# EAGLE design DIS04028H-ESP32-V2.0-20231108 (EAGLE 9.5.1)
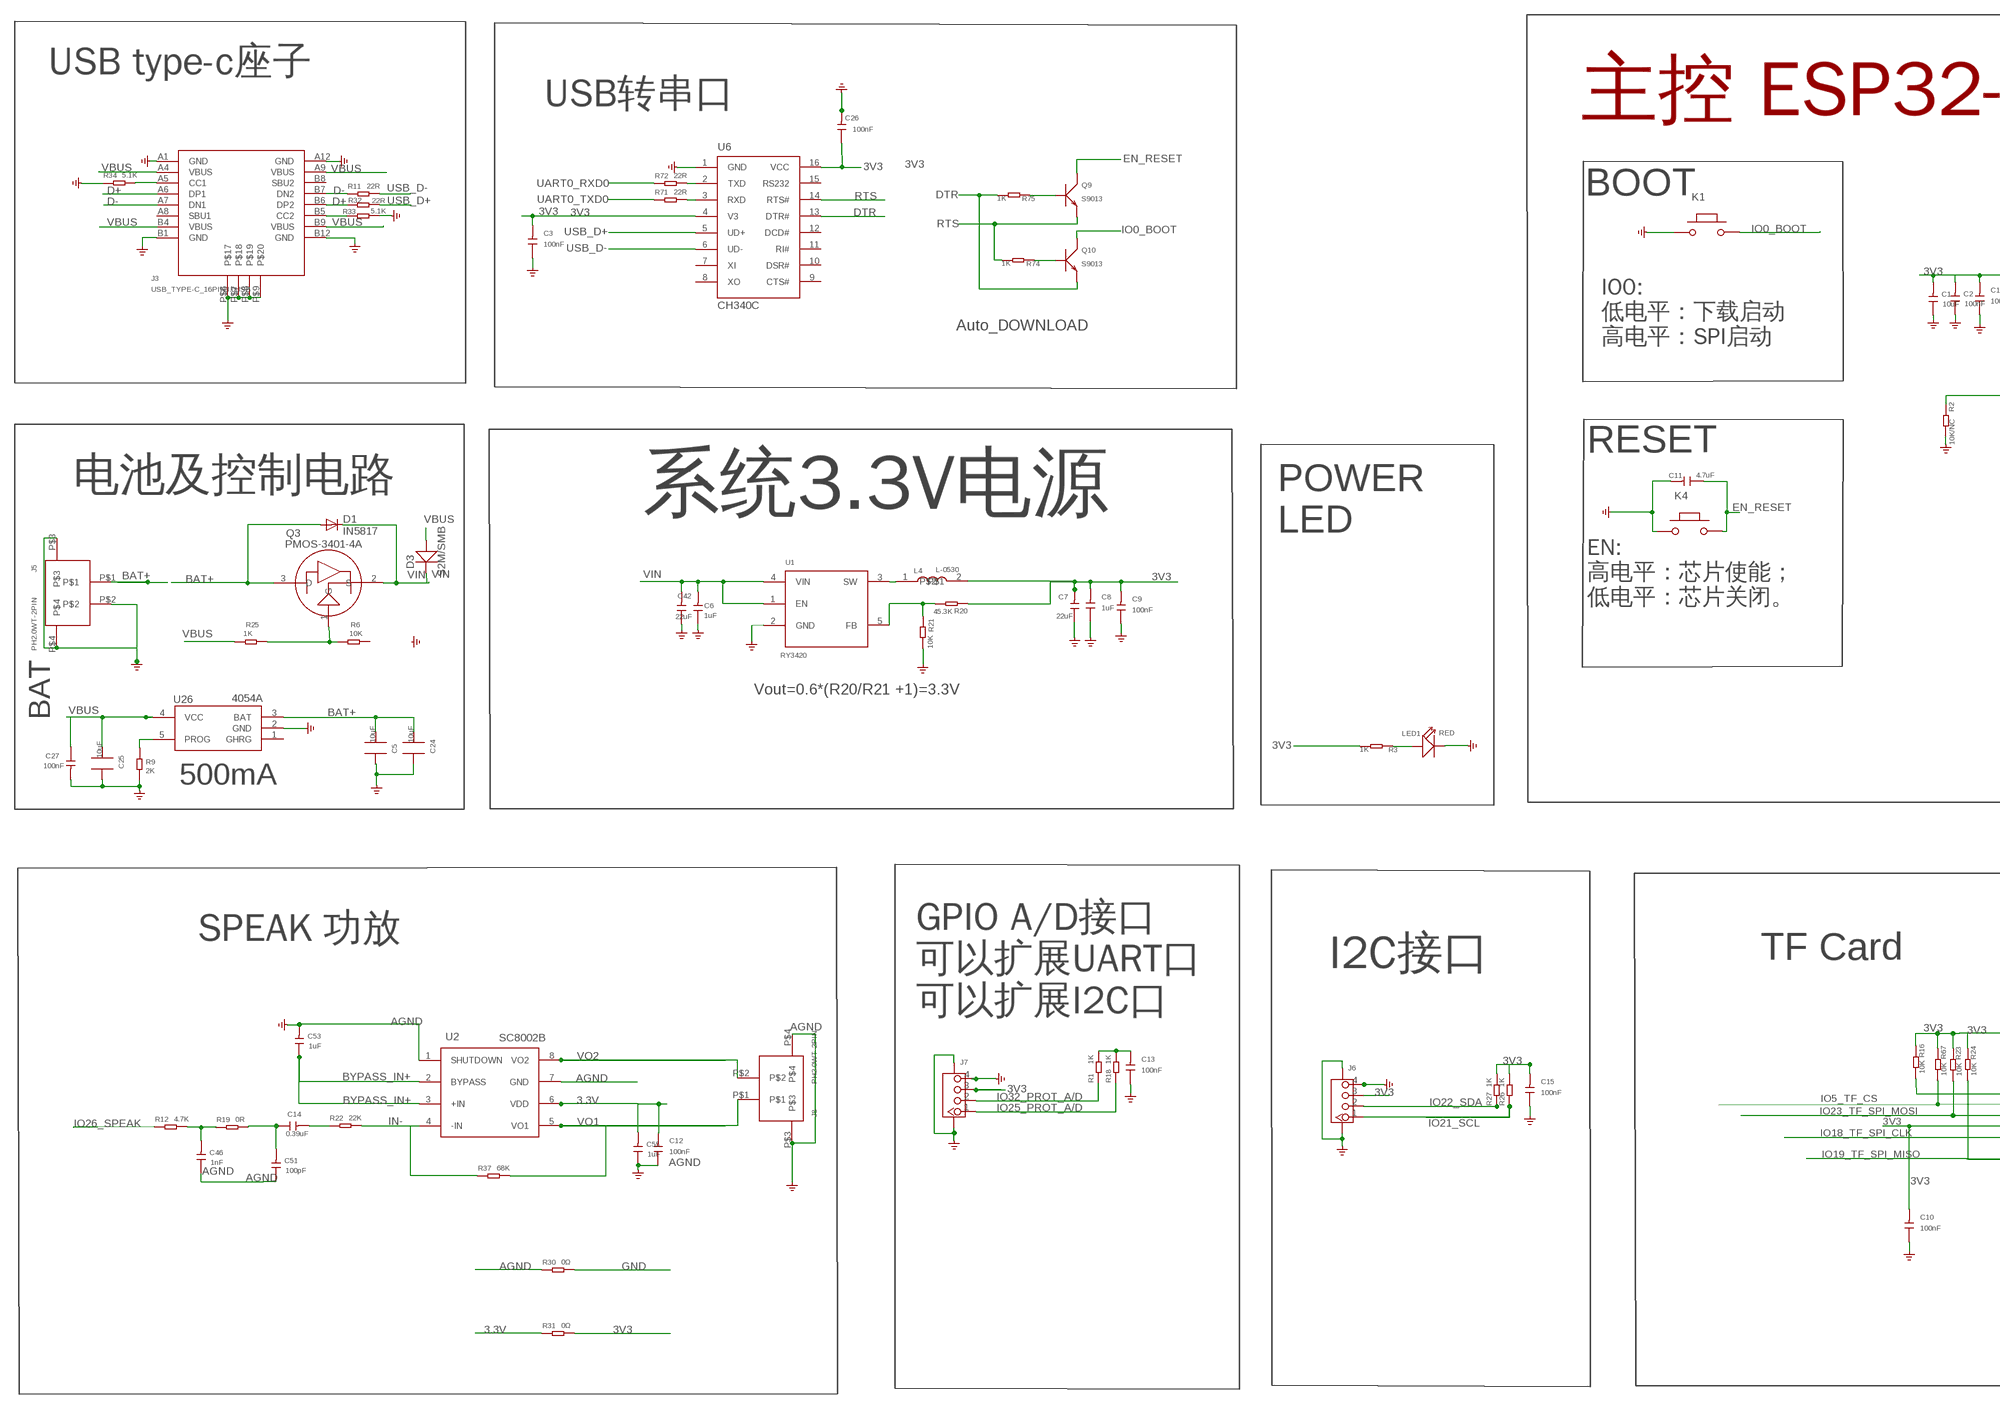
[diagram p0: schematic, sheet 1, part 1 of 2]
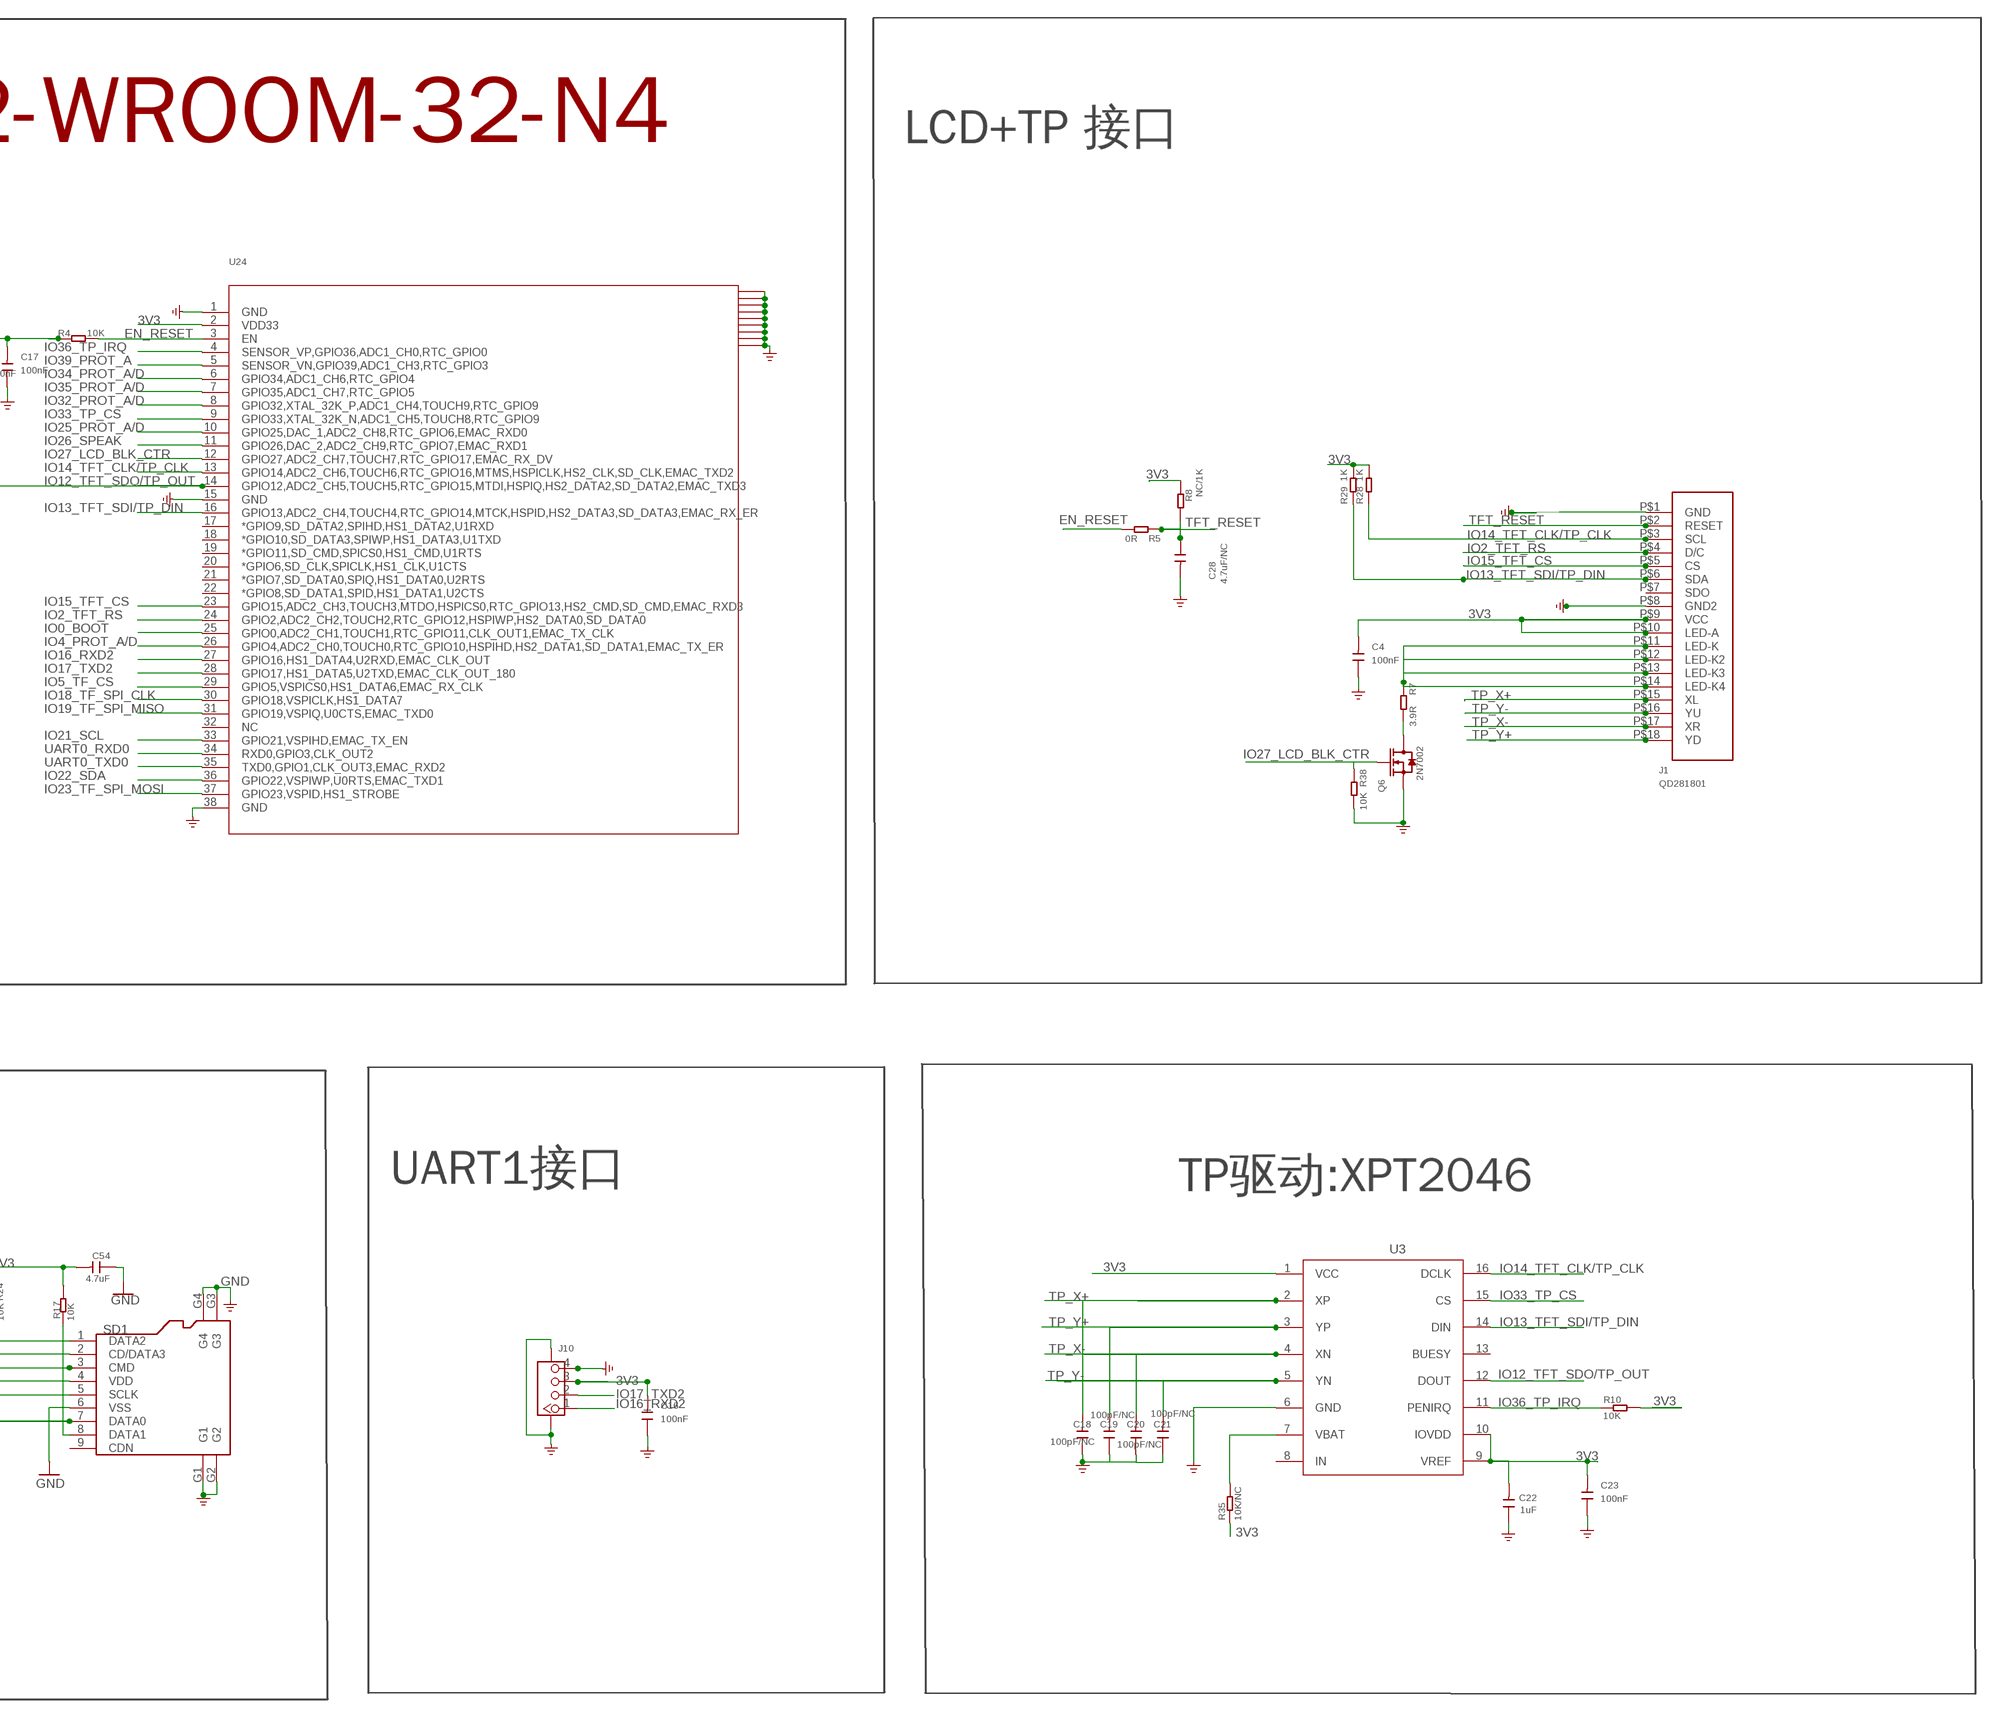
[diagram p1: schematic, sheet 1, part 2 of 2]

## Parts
C1  10uF  DISCRETE_C-0603  [DISCRETE_C0603]
C2  100nF  DISCRETE_C-0603  [DISCRETE_C0603]
C3  100nF  C0603  [0603]
C4  100nF  C0603  [0603]
C5  10uF  C0805_S  [0805_S]
C6  1uF  C0603  [0603]
C7  22uF  C0805  [0805]
C8  1uF  C0603  [0603]
C9  100nF  C0603  [0603]
C10  100nF  C0603  [0603]
C11  4.7uF  C0603  [0603]
C12  100nF  C0603  [0603]
C13  100nF  C0603  [0603]
C14  0.39uF  DISCRETE_C-0603  [DISCRETE_C0603]
C15  100nF  C0603  [0603]
C16  100nF  C0603  [0603]
C17  100nF  C0603  [0603]
C18  100pF/NC  C0603  [0603]
C19  100pF/NC  C0603  [0603]
C20  100pF/NC  C0603  [0603]
C21  100pF/NC  C0603  [0603]
C22  1uF  DISCRETE_C-0603  [DISCRETE_C0603]
C23  100nF  C0603  [0603]
C24  10uF  C0805_S  [0805_S]
C25  10uF  C0805_S  [0805_S]
C26  100nF  C0603  [0603]
C27  100nF  C-0603  [C0603]
C28  4.7uF/NC  C0603  [0603]
C42  22uF  C0805  [0805]
C46  1nF  DISCRETE_C-0603  [DISCRETE_C0603]
C51  100pF  DISCRETE_C-0603  [DISCRETE_C0603]
C53  1uF  DISCRETE_C-0603  [DISCRETE_C0603]
C54  4.7uF  DISCRETE_C-0603  [DISCRETE_C0603]
C55  1uF  DISCRETE_C-0603  [DISCRETE_C0603]
D1  IN5817  DIODE-DO-214AC  [DO-214AC]
D3  S2M/SMB  214ABDO-214AB  [214AB]
J1  QD281801  [QD241801-18PIN*0.8]
J3  USB_TYPE-C_16PIN3.0USB  [KEVIN_3.0TYPEC-SMD]
J5  PH2.0WT-2PIN  [PH2.0WT-2PIN]
J6  CONNECTOR_TWIG-4P-2.0-SMD-FEMALE-REINFORCE90D  [CONNECTOR_4P-SMD-2.0-90D]
J7  CONNECTOR_TWIG-4P-2.0-SMD-FEMALE-REINFORCE90D  [CONNECTOR_4P-SMD-2.0-90D]
J8  PH2.0WT-2PIN  [PH2.0WT-2PIN]
J10  CONNECTOR_TWIG-4P-2.0-SMD-FEMALE-REINFORCE90D  [CONNECTOR_4P-SMD-2.0-90D]
K1  BUTTON  PB157  [157SW]
K4  BUTTON  PB157  [157SW]
L4  L-0530  [CD54_CD54]
LED1  RED  DISCRETE_LED0603  [DISCRETE_LED-0603]
Q3  PMOS-3401-4A  P-MOS-SOT23  [SOT-23]
Q6  2N7002  MOSFET-N'SOT23'  [SOT23]
Q9  S9013  TRANSISTOR-NPN-SOT23  [SOT23@1]
Q10  S9013  TRANSISTOR-NPN-SOT23  [SOT23@1]
R1  1K  DISCRETE_R-0603  [DISCRETE_R0603]
R2  10K/NC  DISCRETE_R-0603  [DISCRETE_R0603]
R3  1K  DISCRETE_R-0603  [DISCRETE_R0603]
R4  10K  R0603  [R0603]
R5  0R  DISCRETE_R-0603  [DISCRETE_R0603]
R6  10K  DISCRETE_R-0603  [DISCRETE_R0603]
R7  3.9R  DISCRETE_R-0603  [DISCRETE_R0603]
R8  NC/1K  DISCRETE_R-0603  [DISCRETE_R0603]
R9  2K  DISCRETE_R-0603  [DISCRETE_R0603]
R10  10K  DISCRETE_R-0603  [DISCRETE_R0603]
R11  22R  DISCRETE_R-0603  [DISCRETE_R0603]
R12  4.7K  DISCRETE_R-0603  [DISCRETE_R0603]
R16  10K  DISCRETE_R-0603  [DISCRETE_R0603]
R17  10K  DISCRETE_R-0603  [DISCRETE_R0603]
R18  1K  DISCRETE_R-0603  [DISCRETE_R0603]
R19  0R  DISCRETE_R-0603  [DISCRETE_R0603]
R20  45.3K  DISCRETE_R-0603  [DISCRETE_R0603]
R21  10K  DISCRETE_R-0603  [DISCRETE_R0603]
R22  22K  DISCRETE_R-0603  [DISCRETE_R0603]
R23  10K  DISCRETE_R-0603  [DISCRETE_R0603]
R24  10K  DISCRETE_R-0603  [DISCRETE_R0603]
R25  1K  DISCRETE_R-0603  [DISCRETE_R0603]
R26  1K  DISCRETE_R-0603  [DISCRETE_R0603]
R27  1K  DISCRETE_R-0603  [DISCRETE_R0603]
R28  1K  DISCRETE_R-0603  [DISCRETE_R0603]
R29  1K  DISCRETE_R-0603  [DISCRETE_R0603]
R30  0Ω  DISCRETE_R-0603  [DISCRETE_R0603]
R31  0Ω  DISCRETE_R-0603  [DISCRETE_R0603]
R32  22R  DISCRETE_R-0603  [DISCRETE_R0603]
R33  5.1K  DISCRETE_R-0603  [DISCRETE_R0603]
R34  5.1K  DISCRETE_R-0603  [DISCRETE_R0603]
R35  10K/NC  DISCRETE_R-0603  [DISCRETE_R0603]
R37  68K  DISCRETE_R-0603  [DISCRETE_R0603]
R38  10K  DISCRETE_R-0603  [DISCRETE_R0603]
R67  10K  DISCRETE_R-0603  [DISCRETE_R0603]
R71  22R  DISCRETE_R-0603  [DISCRETE_R0603]
R72  22R  DISCRETE_R-0603  [DISCRETE_R0603]
R74  1K  DISCRETE_R-0603  [DISCRETE_R0603]
R75  1K  DISCRETE_R-0603  [DISCRETE_R0603]
SD1  HOLDER-MICROSD-9P  [9P-SMD-W/-RING]
U1  RY3420  A_XBJ_HM3420B  [A_XBJ_SOT23-5]
U2  SC8002B  SC8002BSC8002B-SOP8  [AT24C02_SOP8]
U3  XP2046  [XP2046-SSOP16]
U6  CH340C  CH340G  [SOP-16]
U24  ESP32-WROOM-32-N4  [ESP32-WROOM-32-N4]
U26  4054A  [SOP23-5]

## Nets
3.3V: C12.2 C55.2 R31.1 U2.6(VDD)
3V3: C1.2 C2.2 C3.2 C4.2 C7.2 C8.2 C9.2 C10.2 C13.2 C15.2 C16.2 C17.2 C22.2 C23.2 C26.1 C54.2 J1.P$9(VCC) J1.P$10(LED-A) J6.3 J7.3 J10.3 L4.2 R1.2 R3.2 R4.1 R8.2 R10.2 R16.1 R17.1 R18.2 R20.1 R23.1 R24.1 R26.2 R27.2 R28.2 R29.2 R31.2 R35.1 R67.1 SD1.4(VDD) U3.1(VCC) U3.9(VREF) U3.10(IOVDD) U6.4(V3) U6.16(VCC) U24.2(VDD33)
AGND: C12.1 C46.1 C51.1 C53.2 C55.1 J8.P$3 J8.P$4 R30.1 U2.1(SHUTDOWN) U2.7(GND) ; supply symbol labelled GND
BAT+: C5.2 C24.2 D1.A J5.P$1 Q3.3(D) U26.3(BAT)
BYPASS_IN+: C53.1 U2.2(BYPASS) U2.3(+IN)
D+: J3.A6(DP1) J3.B6(DP2) R32.1
D-: J3.A7(DN1) J3.B7(DN2) R11.1
DTR: Q10.2(E) R75.2 U6.13(DTR#)
EN_RESET: C11.1 K4.2 Q9.3(C) R4.2 R5.2 U24.3(EN)
GND: C1.1 C2.1 C3.1 C4.1 C5.1 C6.1 C7.1 C8.1 C9.1 C10.1 C11.2 C13.1 C15.1 C16.1 C17.1 C18.1 C19.1 C20.1 C21.1 C22.1 C23.1 C24.1 C25.1 C26.2 C27.2 C28.2 C42.1 C54.1 J1.P$1(GND) J1.P$8(GND2) J3.A1(GND) J3.A12(GND) J3.B1(GND) J3.B12(GND) J3.P$6 J3.P$7 J3.P$8 J3.P$9 J5.P$2 J5.P$3 J5.P$4 J6.4 J6.SS1 J6.SS2 J7.4 J7.SS1 J7.SS2 J10.4 J10.SS1 J10.SS2 K1.1 K4.1 LED1.- Q6.2(S) R2.2 R9.2 R21.2 R30.2 R33.2 R34.1 R38.2 SD1.6(VSS) SD1.G1 SD1.G2 SD1.G3 SD1.G4 U1.2(GND) U3.6(GND) U6.1(GND) U24.1(GND) U24.15(GND) U24.38(GND) U24.41(GND) U24.42(GND) U24.43(GND) U24.44(GND) U24.45(GND) U24.46(GND) U24.47(GND) U24.48(GND) U24.49(GND) U26.2(GND)
IN-: R22.2 R37.1 U2.4(-IN)
IO0_BOOT: K1.2 Q10.3(C) U24.25(GPIO0,ADC2_CH1,TOUCH1,RTC_GPIO11,CLK_OUT1,EMAC_TX_CLK)
IO2_TFT_RS: J1.P$4(D/C) U24.24(GPIO2,ADC2_CH2,TOUCH2,RTC_GPIO12,HSPIWP,HS2_DATA0,SD_DATA0)
IO4_PROT_A/D: U24.26(GPIO4,ADC2_CH0,TOUCH0,RTC_GPIO10,HSPIHD,HS2_DATA1,SD_DATA1,EMAC_TX_ER)
IO5_TF_CS: R67.2 SD1.2(CD/DATA3) U24.29(GPIO5,VSPICS0,HS1_DATA6,EMAC_RX_CLK)
IO12_TFT_SDO/TP_OUT: R2.1 U3.12(DOUT) U24.14(GPIO12,ADC2_CH5,TOUCH5,RTC_GPIO15,MTDI,HSPIQ,HS2_DATA2,SD_DATA2,EMAC_TXD3)
IO13_TFT_SDI/TP_DIN: J1.P$6(SDA) R29.1 U3.14(DIN) U24.16(GPIO13,ADC2_CH4,TOUCH4,RTC_GPIO14,MTCK,HSPID,HS2_DATA3,SD_DATA3,EMAC_RX_ER)
IO14_TFT_CLK/TP_CLK: J1.P$3(SCL) R28.1 U3.16(DCLK) U24.13(GPIO14,ADC2_CH6,TOUCH6,RTC_GPIO16,MTMS,HSPICLK,HS2_CLK,SD_CLK,EMAC_TXD2)
IO15_TFT_CS: J1.P$5(CS) U24.23(GPIO15,ADC2_CH3,TOUCH3,MTDO,HSPICS0,RTC_GPIO13,HS2_CMD,SD_CMD,EMAC_RXD3)
IO16_RXD2: J10.1 U24.27(GPIO16,HS1_DATA4,U2RXD,EMAC_CLK_OUT)
IO17_TXD2: J10.2 U24.28(GPIO17,HS1_DATA5,U2TXD,EMAC_CLK_OUT_180)
IO18_TF_SPI_CLK: SD1.5(SCLK) U24.30(GPIO18,VSPICLK,HS1_DATA7)
IO19_TF_SPI_MISO: R24.2 SD1.7(DATA0) U24.31(GPIO19,VSPIQ,U0CTS,EMAC_TXD0)
IO21_SCL: J6.1 R26.1 U24.33(GPIO21,VSPIHD,EMAC_TX_EN)
IO22_SDA: J6.2 R27.1 U24.36(GPIO22,VSPIWP,U0RTS,EMAC_TXD1)
IO23_TF_SPI_MOSI: R23.2 SD1.3(CMD) U24.37(GPIO23,VSPID,HS1_STROBE)
IO25_PROT_A/D: J7.1 R18.1 U24.10(GPIO25,DAC_1,ADC2_CH8,RTC_GPIO6,EMAC_RXD0)
IO26_SPEAK: R12.1 U24.11(GPIO26,DAC_2,ADC2_CH9,RTC_GPIO7,EMAC_RXD1)
IO27_LCD_BLK_CTR: Q6.1(G) R38.1 U24.12(GPIO27,ADC2_CH7,TOUCH7,RTC_GPIO17,EMAC_RX_DV)
IO32_PROT_A/D: J7.2 R1.1 U24.8(GPIO32,XTAL_32K_P,ADC1_CH4,TOUCH9,RTC_GPIO9)
IO33_TP_CS: U3.15(CS) U24.9(GPIO33,XTAL_32K_N,ADC1_CH5,TOUCH8,RTC_GPIO9)
IO34_PROT_A/D: U24.6(GPIO34,ADC1_CH6,RTC_GPIO4)
IO35_PROT_A/D: U24.7(GPIO35,ADC1_CH7,RTC_GPIO5)
IO36_TP_IRQ: R10.1 U3.11(PENIRQ) U24.4(SENSOR_VP,GPIO36,ADC1_CH0,RTC_GPIO0)
IO39_PROT_A: U24.5(SENSOR_VN,GPIO39,ADC1_CH3,RTC_GPIO3)
N$1: LED1.+ R3.1
N$2: Q6.3(D) R7.2
N$3: C46.2 R12.2 R19.1
N$4: R35.2 U3.7(VBAT)
N$6: R9.1 U26.5(PROG)
N$8: L4.1 U1.3(SW)
N$12: J1.P$11(LED-K) J1.P$12(LED-K2) J1.P$13(LED-K3) J1.P$14(LED-K4) R7.1
N$14: J3.B5(CC2) R33.1
N$16: J3.A5(CC1) R34.2
N$17: Q3.1(G) R6.2 R25.1
N$20: R20.2 R21.1 U1.5(FB)
N$26: C14.1 C51.2 R19.2
N$29: C14.2 R22.1
N$32: Q9.1(B) R75.1
N$38: Q10.1(B) R74.1
N$40: R72.2 U6.2(TXD)
N$42: R71.2 U6.3(RXD)
N$47: R16.2 SD1.1(DATA2)
N$48: R17.2 SD1.8(DATA1)
RTS: Q9.2(E) R74.2 U6.14(RTS#)
TFT_RESET: C28.1 J1.P$2(RESET) R5.1 R8.1
TP_X+: C18.2 J1.P$15(XL) U3.2(XP)
TP_X-: C20.2 J1.P$17(XR) U3.4(XN)
TP_Y+: C19.2 J1.P$18(YD) U3.3(YP)
TP_Y-: C21.2 J1.P$16(YU) U3.5(YN)
UART0_RXD0: R72.1 U24.34(RXD0,GPIO3,CLK_OUT2)
UART0_TXD0: R71.1 U24.35(TXD0,GPIO1,CLK_OUT3,EMAC_RXD2)
USB_D+: R32.2 U6.5(UD+)
USB_D-: R11.2 U6.6(UD-)
VBUS: C25.2 C27.1 D3.1(+) J3.A4(VBUS) J3.A9(VBUS) J3.B4(VBUS) J3.B9(VBUS) R25.2 U26.4(VCC)
VIN: C6.2 C42.2 D1.C D3.2(-) Q3.2(S) U1.1(EN) U1.4(VIN)
VO1: J8.P$1 R37.2 U2.5(VO1)
VO2: J8.P$2 U2.8(VO2)
Unconnected: J1.P$7(SDO) J3.A8(SBU1) J3.B8(SBU2) R6.1 SD1.9(CDN) U3.8(IN) U3.13(BUESY) U6.7(XI) U6.8(XO) U6.9(CTS#) U6.10(DSR#) U6.11(RI#) U6.12(DCD#) U6.15(RS232) U24.17(*GPIO9,SD_DATA2,SPIHD,HS1_DATA2,U1RXD) U24.18(*GPIO10,SD_DATA3,SPIWP,HS1_DATA3,U1TXD) U24.19(*GPIO11,SD_CMD,SPICS0,HS1_CMD,U1RTS) U24.20(*GPIO6,SD_CLK,SPICLK,HS1_CLK,U1CTS) U24.21(*GPIO7,SD_DATA0,SPIQ,HS1_DATA0,U2RTS) U24.22(*GPIO8,SD_DATA1,SPID,HS1_DATA1,U2CTS) U24.32(NC) U26.1(GHRG)

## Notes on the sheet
- USB type-c座子
- USB转串口 | 主控 ESP32-WROOM-32-N4 | LCD+TP 接口
- BOOT
- Auto_DOWNLOAD
- IO0:
  低电平：下载启动
  高电平：SPI启动
- RESET
- 电池及控制电路
- 系统3.3V电源
- POWER
  LED
- EN:
  高电平：芯片使能；
  低电平：芯片关闭。
- Vout=0.6*(R20/R21 +1)=3.3V
- BAT
- 500mA
- SPEAK 功放
- I2C接口 | TF Card | UART1接口
- TP驱动:XPT2046
- GPIO A/D接口
  可以扩展UART口
  可以扩展I2C口

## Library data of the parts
C1 C2 C14 C22 C46 C51 C53 C55 = A_xbj:DISCRETE_C*: Ceramic Capacitors
C3 C4 C6 C8-C13 C15-C21 C23 C26 C28 = A_xbj:C0603
C5 C24 C25 = CPT_SMD:C0805
C7 C42 = A_xbj:C0805
C27 = discrete:C*: Ceramic Capacitors
C54 = A9G:DISCRETE_C*: Ceramic Capacitors
D1 = diode:DIODE-: DIODE
D3 = DO-214AB:214AB: 214AB
J1 = cooper:QD281801
J3 = WZ3532R024-ESP32-V0.1-20221226:USB_TYPE-C_16PIN
J5 J8 = cooper:PH2.0WT-2PIN
J6 J7 J10 = A_xbj:CONNECTOR_TWIG-4P-2.0-SMD-FEMALE-REINFORCE
K1 K4 = MySMD:PB157
L4 = WZ2432R028-ESP32-V1.2-20231108:L-0530
LED1 = A_xbj:DISCRETE_LED*
Q3 = DFN8:P-MOS-SOT23
Q6 = discrete:MOSFET-N: IRLL014: http://www.vishay.com/docs/91319/sihll014.pdf
Q9 Q10 = discrete:TRANSISTOR-NPN*: NPN audion
R1-R3 R5 R7 R8 R11 R12 R16-R24 R26-R34 R37 R38 R67 R71 R72 R74 R75 = Crowtail-_LED-V2.0-20190615-01:DISCRETE_R*
R4 = A_xbj:R0603
R6 R9 R10 R25 R35 = A9G:DISCRETE_R*
SD1 = Connector:HOLDER-MICROSD-9P
U1 = CrowBot_-V1.0-20220525:A_XBJ_HM3420B
U2 = cooper:SC8002B
U3 = cooper:XP2046
U6 = A_xbj:CH340G
U24 = cooper:ESP32-WROOM-32-N4
U26 = DFN8:4054A

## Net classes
0 default: width 0.152 mm, drill 0.305 mm, clearance 0.203 mm

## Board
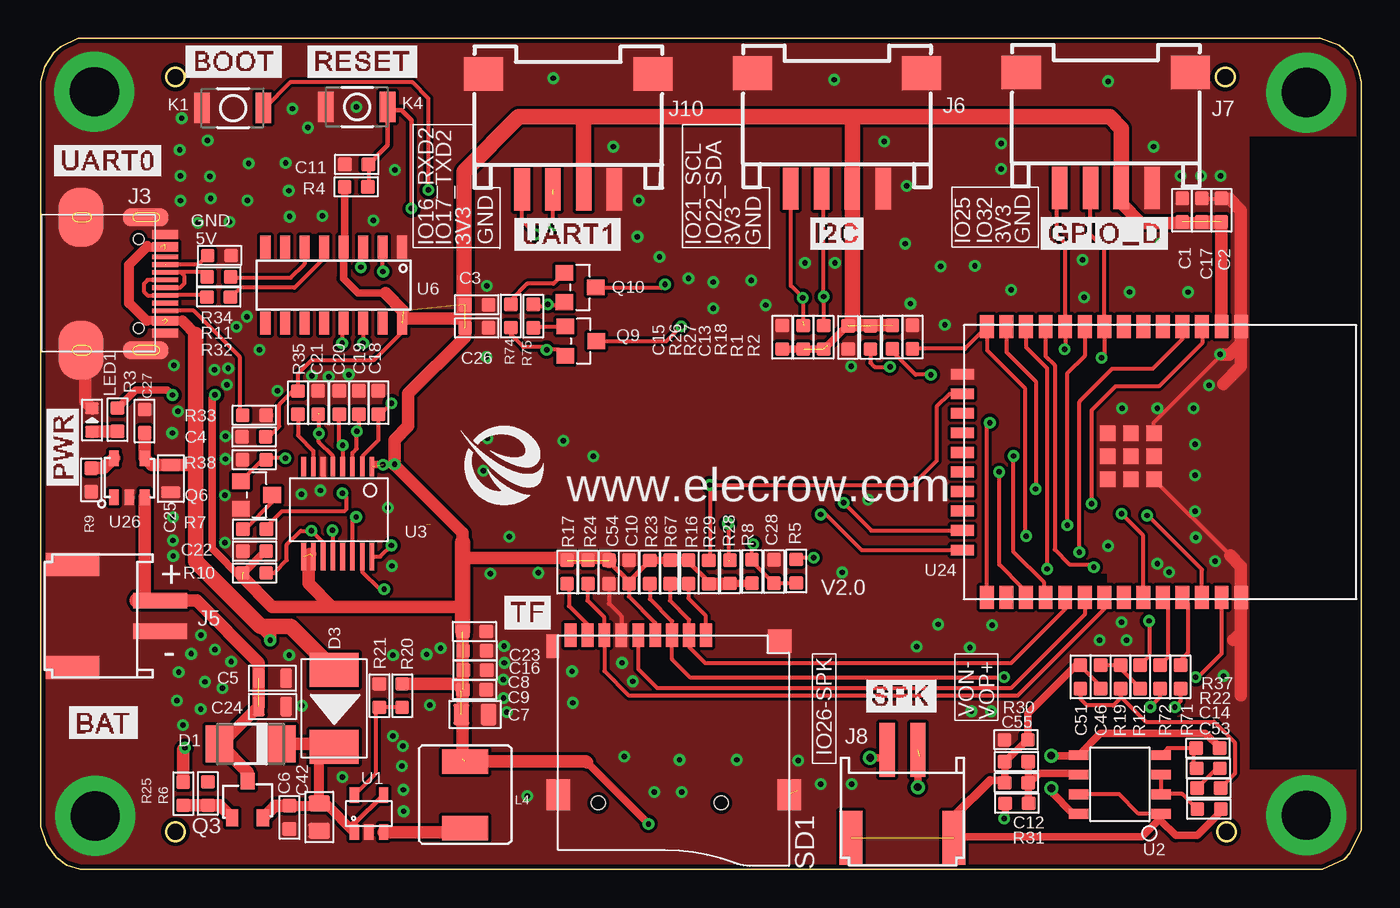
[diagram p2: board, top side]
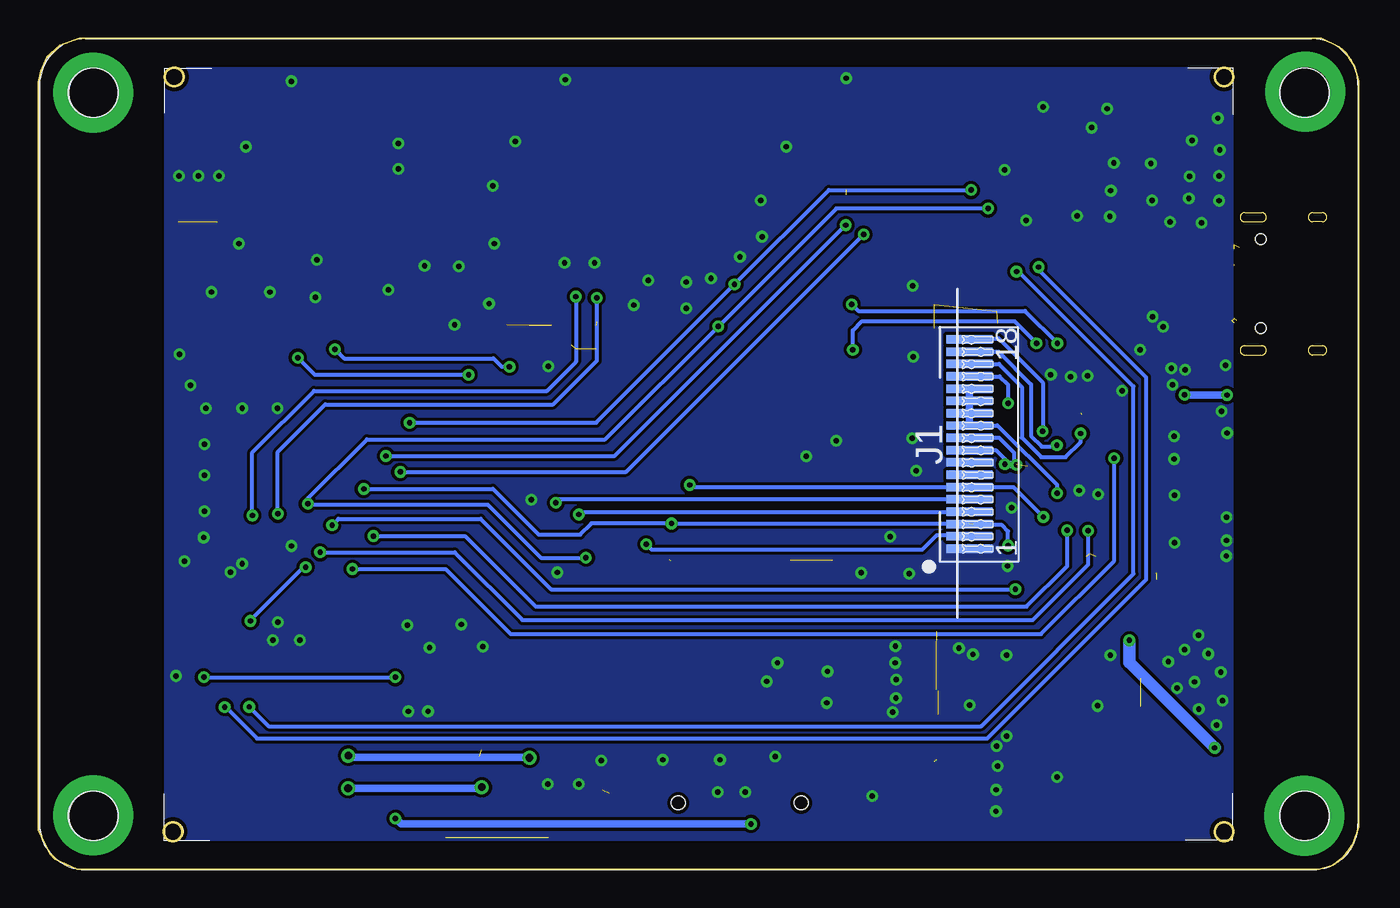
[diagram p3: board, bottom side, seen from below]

Size 85.8 x 54 mm. Coordinates in mm from the lower left corner, seen from the top.
Outline: 83.16,54 84.38,53.56 85.25,52.77 85.65,51.88 85.8,51.16 85.8,2.55 85.06,1.03 84.71,0.66 83.28,0 2.57,0 1.7,0.28 1.01,0.77 0.38,1.61 0,2.75 0,51.24 0.27,52.16 0.86,53.08 1.3,53.47 2.44,54 83.16,54
Outline: circle at 76.98,51.5 radius 0.59
Outline: circle at 8.77,2.44 radius 0.59
Outline: circle at 77.06,2.44 radius 0.59
Outline: circle at 8.77,51.5 radius 0.59
Copper layers (1*16): Top 0.035mm / dielectric 1.5mm / Bottom 0.035mm
Design rules "default *": minimum track width 6mil, minimum drill 0.35mm, track to track 6mil, track to pad 4mil, pad to pad 4mil, via to via 6mil, smd to smd 6mil, copper to edge 10mil, drill to drill 10mil, minimum pad ring 10mil, minimum via ring 8mil, stop-mask expansion 4mil, vias tented up to drill 100mil, thermal gap 0mil
tRestrict: area 21.1,130.4 to 30.9,149.4
bRestrict: area 21.1,130.4 to 30.9,149.4

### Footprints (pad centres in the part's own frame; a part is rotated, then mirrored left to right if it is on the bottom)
DISCRETE_C0603 = smd 0.889 x 0.889: 1 -0.762,0; 2 0.762,0
0603 = smd 0.889 x 0.889: 1 -0.762,0; 2 0.762,0
0805_S = smd 0.762 x 1.27: 1 -0.889,0; 2 0.889,0
0805 = smd 1.016 x 1.397: 1 -0.889,0; 2 0.889,0
C0603 = smd 0.889 x 0.889: 1 -0.762,0; 2 0.762,0
DO-214AC = smd 1.8 x 2.4: A 2.025,0; C -2.025,0
214AB = smd 2.2 x 3.2: 1 -2.5,0; 2 2.5,0
QD241801-18PIN*0.8 = smd 0.55 x 3: P$1 -6.789,-1.538; P$2 -5.989,-1.538; P$3 -5.189,-1.538; P$4 -4.389,-1.538; P$5 -3.589,-1.538; P$6 -2.789,-1.538; P$7 -1.989,-1.538; P$8 -1.189,-1.538; P$9 -0.389,-1.538; P$10 0.411,-1.538; P$11 1.211,-1.538; P$12 2.011,-1.538; P$13 2.811,-1.538; P$14 3.611,-1.538; P$15 4.411,-1.538; P$16 5.211,-1.538; P$17 6.011,-1.538; P$18 6.811,-1.538
KEVIN_3.0TYPEC-SMD = smd 0.3 x 1.7: A1 -3.35,0.5; A4 -2.55,0.5; A5 -1.25,0.5; A6 -0.25,0.5; A7 0.25,0.5; A8 1.25,0.5; A9 2.55,0.5; A12 3.35,0.5; B1 3.05,0.5; B4 2.25,0.5; B5 1.75,0.5; B6 0.75,0.5; B7 -0.75,0.5; B8 -1.75,0.5; B9 -2.25,0.5; B12 -3.05,0.5 | smd 1.143 x 2.921: P$6 -4.318,-0.762; P$7 4.318,-0.762 | smd 3.81 x 2.921: P$8 -4.318,-4.953; P$9 4.318,-4.953 | hole 0.68: -2.89,-1.22; 2.89,-1.22
PH2.0WT-2PIN = smd 1 x 3.5: P$1 -1,0; P$2 1,0 | smd 1.5 x 3.5: P$3 -3.35,-5.7; P$4 3.35,-5.7
CONNECTOR_4P-SMD-2.0-90D = smd 1.01 x 2.74: 1 -3,-0.1; 2 -1,-0.1; 3 1,-0.1; 4 3,-0.1 | smd 2.54 x 2.184: SS1 -5.5,7.4; SS2 5.5,7.4
157SW = smd 1.016 x 1.981: 1 0,0; 2 4,0
CD54_CD54 = smd 3 x 1.6: 1 0,2.159; 2 0,-2.159
DISCRETE_LED-0603 = smd 0.762 x 0.889: + -0.762,0; - 0.762,0
SOT-23 = smd 1.1 x 0.8: 1 1.2,-1; 2 1.2,1 | smd 1.1 x 0.9: 3 -1.2,0
SOT23 = smd 1.016 x 1.143: 1 -0.889,-1.016; 2 0.889,-1.016; 3 0,1.016
SOT23@1 = smd 1.016 x 1.143: 1 -0.95,-1.016; 2 0.95,-1.016; 3 0,1.016
DISCRETE_R0603 = smd 0.889 x 0.889: 1 -0.762,0; 2 0.762,0
R0603 = smd 0.889 x 0.889: 1 -0.762,0; 2 0.762,0
9P-SMD-W/-RING = smd 1.524 x 0.762: 1 0,4.4; 2 0,3.3; 3 0,2.2; 4 0,1.1; 5 0,0; 6 0,-1.1; 7 0,-2.2; 8 0,-3.3; 9 0,-4.4 | smd 1.524 x 0.8: G1 0.7,-5.546 | smd 2.032 x 1.524: G2 10.373,-5.2; G3 10.373,9.8 | smd 1.524 x 1.524: G4 0.392,9.181 | hole 0.889: 10.9,-2.6; 10.9,5.4
A_XBJ_SOT23-5 = smd 0.6 x 1: 1 -0.95,-1.2; 2 0,-1.2; 3 0.95,-1.2; 4 0.95,1.2; 5 -0.95,1.2
AT24C02_SOP8 = smd 0.635 x 1.27: 1 -1.905,-2.667; 2 -0.635,-2.667; 3 0.635,-2.667; 4 1.905,-2.667; 5 1.905,2.667; 6 0.635,2.667; 7 -0.635,2.667; 8 -1.905,2.667
XP2046-SSOP16 = smd 0.305 x 1.27: 1 -2.54,-2.54; 2 -1.905,-2.54; 3 -1.27,-2.54; 4 -0.635,-2.54; 5 0,-2.54; 6 0.635,-2.54; 7 1.27,-2.54; 8 1.905,-2.54 | smd 0.305 x 1.778: 9 1.905,3.302; 10 1.27,3.302; 11 0.635,3.302; 12 0,3.302; 13 -0.635,3.302; 14 -1.27,3.302; 15 -1.905,3.302; 16 -2.54,3.302
SOP-16 = smd 0.66 x 1.5: 1 -4.445,-2.475; 2 -3.175,-2.475; 3 -1.905,-2.475; 4 -0.635,-2.475; 5 0.635,-2.475; 6 1.905,-2.475; 7 3.175,-2.475; 8 4.445,-2.475; 9 4.445,2.475; 10 3.175,2.475; 11 1.905,2.475; 12 0.635,2.475; 13 -0.635,2.475; 14 -1.905,2.475; 15 -3.175,2.475; 16 -4.445,2.475
ESP32-WROOM-32-N4 = smd 1.5 x 0.9: 1 -8.898,6.761; 2 -8.898,5.491; 3 -8.898,4.221; 4 -8.898,2.951; 5 -8.898,1.681; 6 -8.898,0.411; 7 -8.898,-0.859; 8 -8.898,-2.129; 9 -8.898,-3.399; 10 -8.898,-4.669; 11 -8.898,-5.939; 12 -8.898,-7.209; 13 -8.898,-8.479; 14 -8.898,-9.749; 25 8.702,-9.749; 26 8.702,-8.479; 27 8.702,-7.209; 28 8.702,-5.939; 29 8.702,-4.669; 30 8.702,-3.399; 31 8.702,-2.129; 32 8.702,-0.859; 33 8.702,0.411; 34 8.702,1.681; 35 8.702,2.951; 36 8.702,4.221; 37 8.702,5.491; 38 8.702,6.761 | smd 0.7 x 1.5: 15 -5.808,-11.349; 16 -4.538,-11.349; 17 -3.268,-11.349; 18 -1.998,-11.349; 19 -0.728,-11.349; 20 0.542,-11.349; 21 1.812,-11.349; 22 3.082,-11.349; 23 4.352,-11.349; 24 5.622,-11.349 | smd 1 x 1: 41 -0.484,-0.402; 42 1.016,-0.402; 43 -1.984,-0.402; 44 -1.984,-1.902; 45 -0.484,-1.902; 46 1.016,-1.902; 47 1.016,1.098; 48 -0.484,1.098; 49 -1.984,1.098
SOP23-5 = smd 1 x 0.635: 1 -1.27,1; 2 -1.27,0; 3 -1.27,-1; 4 1.27,-1; 5 1.27,1

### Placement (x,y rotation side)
C1  74.18,42.84 270 top
C2  76.72,42.84 270 top
C3  28.34,36.69 180 top
C4  13.86,28.11 0 top
C5  15.06,12.42 180 top
C6  16.17,3.38 90 top
C7  28.22,10.06 180 top
C8  28.22,12.95 180 top
C9  28.2,11.68 180 top
C10  38.23,19.33 270 top
C11  20.54,45.81 180 top
C12  63.41,5.63 0 top
C13  52.47,34.57 90 top
C14  75.9,5.28 180 top
C15  48.18,34.58 270 top
C16  28.22,14.22 180 top
C17  75.45,42.84 270 top
C18  21.94,30.33 270 top
C19  20.67,30.33 270 top
C20  19.4,30.33 270 top
C21  18.03,30.33 270 top
C22  13.9,20.68 0 top
C23  28.19,15.46 180 top
C24  15.07,10.58 180 top
C25  8.46,25.4 90 top
C26  28.34,35.19 0 top
C27  6.76,29.13 90 top
C28  47.65,19.35 90 top
C42  18.11,3.4 90 top
C46  68.88,12.51 90 top
C51  67.57,12.51 270 top
C53  75.92,3.91 0 top
C54  36.93,19.33 90 top
C55  63.41,7 0 top
D1  13.64,8.15 180 top
D3  19.07,10.46 270 top
J1  26.84,27.63 90 bottom
J3  7.58,38.05 270 top
J5  7.77,16.47 270 top
J6  51.74,44.34 0 top
J7  69.21,44.39 0 top
J8  56.01,7.76 0 top
J10  34.28,44.29 0 top
K1  10.48,49.48 0 top
K4  18.54,49.55 0 top
L4  27.59,4.85 180 top
LED1  3.34,29.2 90 top
Q3  13.45,4.53 270 top
Q6  14.03,24.33 270 top
Q9  35.1,34.33 270 top
Q10  35.05,37.82 270 top
R1  55.35,34.6 90 top
R2  56.65,34.6 90 top
R3  5,29.23 90 top
R4  20.51,44.36 0 top
R5  49.1,19.38 90 top
R6  10.86,4.93 270 top
R7  13.91,22.1 180 top
R8  46.23,19.35 270 top
R9  3.28,25.31 270 top
R10  13.89,19.26 180 top
R11  11.58,38.51 0 top
R12  71.44,12.51 270 top
R16  42.1,19.33 270 top
R17  34.21,19.33 270 top
R18  53.92,34.57 90 top
R19  70.17,12.51 270 top
R20  23.49,11.29 270 top
R21  22.01,11.29 90 top
R22  75.87,6.56 180 top
R23  39.59,19.32 270 top
R24  35.57,19.33 270 top
R25  9.26,4.91 90 top
R26  49.55,34.58 270 top
R27  50.88,34.58 270 top
R28  44.8,19.34 270 top
R29  43.42,19.31 270 top
R30  63.39,8.42 180 top
R31  63.44,4.29 180 top
R32  11.57,37.19 0 top
R33  13.89,29.51 0 top
R34  11.62,39.89 180 top
R35  16.72,30.33 270 top
R37  75.85,7.87 0 top
R38  13.89,26.63 180 top
R67  40.92,19.33 270 top
R71  74.07,12.51 270 top
R72  72.74,12.51 270 top
R74  30.55,35.97 270 top
R75  32.01,35.95 90 top
SD1  38.83,15.22 270 top
U1  21.33,3.62 0 top
U2  70.13,5.52 90 top
U3  18.99,23.63 180 top
U6  19.05,37.96 180 top
U24  71.24,26.37 270 top
U26  5.76,25.46 90 top
U$2  [2.8板框]  not placed on the board
U$30  [ELECROW-NEW]  27.26,23.67 0 top

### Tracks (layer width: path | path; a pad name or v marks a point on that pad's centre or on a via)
1
  cutout Top: 17.5,41.25 18.05,41.25 18.05,39.7 17.5,39.7
  cutout Top: 67.7,18.6 67.7,19.15 69.25,19.15 69.25,18.6
  cutout Top: 73.65,11.3 73.1,11.3 73.1,12.85 73.65,12.85
  cutout Top: 35.2,17.45 34.65,17.45 34.65,19 35.2,19
3.3V
  Top 0.254: R31.1 64.2,5.54 | 64.2,5.6 C12.2
  Top 0.5: U2.6 67.38,6.23 64.89,6.23 64.2,5.54 | R31.1 64.2,5.6 | C12.2 C55.2
3V3  (via drill 0.35)  (21 unrouted)
  Top 0.203: 27.33,11.58 C9.2 27.46,11.71 | C8.2 27.43,12.93
  Top 0.254: C10.2 38.23,17.72 39.93,16.02 SD1.4 | v62.6,3.3 62.68,3.38 | 14.6,20.68 C22.2 | 23.81,35.8 U6.16 23.5,34.93 21.68,33.11 17.61,33.11 16.72,32.22 R35.1 16.39,31.09 15.5,30.2 15.5,28.78 14.82,28.11 C4.2 | R16.1 R67.1
  Top 0.3: 36.93,19.99 38.23,18.7 39.59,20.06 | 43.42,18.67 42.1,19.98
  Top 0.5: 62.68,3.38 R31.2 | v39.5,2.95 35.49,6.96 | C23.2 27.43,15.61 | R4.1 19.75,40.5 U6.4 19.69,38.4 20.63,37.45 22.4,37.45 | C54.2 36.93,19.99 | 39.59,20.06 R23.1 R16.1 42.1,19.98 | C10.2 38.23,18.7 | 43.42,18.67 R29.2 | 52.74,35.65 52.47,35.38 51.16,34.07 | C15.2 R27.2 | 22.97,26.32 21.68,26.32 21.7,26.3 v22.25,26.3 | 13.13,18.86 11.13,20.85 11.13,30.63 v11.33,30.83 | v8.57,30.83 8.23,31.16 6.17,31.16 R3.2 | 13.18,19.26 14.6,20.68 | 44.92,18.69 R28.2 46.21,18.58 R8.2
  Top 0.8: 27.43,7.16 C23.2 | C9.2 27.07,12.05 R20.1 | 27.51,35.8 23.81,35.8 | J6.3 52.79,44.29 | J7.3 70.22,43.29 71.5,42 76.64,42 C2.2 | U24.2 76.73,41.82 76.47,42.08 C17.2 | 23.55,36.3 22.4,37.45 | R1.2 52.49,35.36 52.47,35.38 | 36.87,20.15 36.77,20.25 27.43,20.25 | R29.2 44.77,18.55 R28.2 | 27.43,21.23 27.43,21.85 22.97,26.32 | v23,26.32 23,27.92 23.89,28.81 23.89,30.92 27.58,34.6 C26.1 | 27.43,17.07 18.92,17.07 | 18.92,17.07 17.42,18.57 17.42,20.42 17.51,20.5 | R10.2 13.13,19 15.06,17.07 18.92,17.07 | 35.49,6.96 35.44,7.01 L4.2
  Top 1: C23.2 27.43,17.07 27.43,20.25 27.43,21.23 | C54.2 36.87,20.15 | 27.51,35.8 27.51,45.36 31.05,48.9 35.5,48.9 | 35.5,48.9 52.65,48.9 | 52.65,48.9 69.47,48.9 70.22,48.15 J7.3 | 52.74,35.65 J6.3 52.74,48.81 52.65,48.9 | 35.5,48.9 35.28,48.68 J10.3
  Bottom 0.254: J1.P$10 23.37,28.04 22.41,27.08 22.41,26.32 v23,26.32 23,26.65 23.59,27.24 J1.P$9
  Bottom 0.5: v62.6,3.3 62.25,2.95 v39.5,2.95 | v23,26.32 22.27,26.32 v22.25,26.3 | v11.33,30.83 v8.57,30.83
AGND  (1 unrouted)
  Top 0.254: C46.1 68.88,11.9 67.57,13.21 C51.1 67.57,13.32 | 64.01,8.42 R30.1 64.15,8.45 64.14,8.45 | C53.2 76.69,3.74 | U2.7 67.48,4.9 70.05,4.9 71.34,3.61 U2.1 72.79,3.35 72.79,3.16 | J8.P$4 59.36,3.44
  Top 0.5: 64.15,8.45 64.15,10.15 67.27,13.27 C51.1 | 64.14,8.45 62.7,7.01 C55.1 C12.1 62.5,5.78 61.7,5.78 | 76.69,3.74 75.15,2.2 73.75,2.2 72.79,3.16 | J8.P$4 59.4,2.1 71.54,2.1 72.79,3.35
  Top 0.58: 61.7,5.78 59.36,3.44
BAT+  (1 unrouted)
  Top 0.8: U26.3 6.76,17.48 6.76,17.47 | J5.P$1 10.14,17.47 14.18,13.43 C24.2 11.74,8.15 D1.A 13.45,6.32 Q3.3
  Top 1: J5.P$1 6.76,17.47 6.27,17.47
BYPASS_IN+
  Top 0.254: U2.3 U2.2 72.81,4.9 74.17,4.9 C53.1
D+
  Top 0.254: R32.1 10.81,37.21 10.7,37.32 8.1,37.32 J3.B6 6.95,37.3 6.7,37.55 6.7,38.05 6.96,38.3 J3.A6
D-
  Top 0.254: R11.1 10.82,38.62 10.63,38.81 J3.B7 9.08,38.8 9.09,38.81 9.35,38.55 9.35,38.1 9.05,37.8 J3.A7
DTR  (via drill 0.35)
  Top 0.254: Q10.2 33.82,36.65 33.03,36.65 v32.96,36.73 32.81,36.58 32.14,36.58 R75.2 | U6.13 19.59,35.39 v19.59,34.19
  Bottom 0.254: v32.96,36.73 32.52,36.29 21.69,36.29 v19.59,34.19
EN_RESET  (via drill 0.35)
  Top 0.254: U24.3 75.47,35.26 75.47,34.2 72.66,31.39 69.84,31.39 68.3,29.85 v68.3,23.75 | C11.1 21.3,44.39 R4.2 | Q9.3 40.66,34.33 v41.62,35.29 | v50.22,20.25 49.21,20.25 R5.2
  Top 0.3: v24.1,42.95 24.1,48.7 23.45,49.35 22.74,49.35 | C11.1 22.56,47.07 22.56,48.96 22.26,49.26 K4.2
  Top 0.5: 22.74,49.35 K4.2
  Bottom 0.254: v24.1,42.95 33.95,42.95 v41.62,35.29 48.97,27.94 64.45,27.94 68.3,24.09 v68.3,23.75 68.25,23.7 56.6,23.7 53.15,20.25 v50.22,20.25
GND  (via drill 0.35, 3.2 pad 5.2)  (1 unrouted)
  Top 0.203: C42.1 17.72,2.9 | C7.1 29.26,9.91 | C9.1 29.11,11.53 | 28.96,12.93 C8.1
  Top 0.254: C54.1 36.93,17.27 37.73,16.47 SD1.6 | 49.13,5.14 48.4,4.41 | 48.72,4.93 SD1.G3 | 62.48,8.57 R30.2 | U24.49 72.34,29.04 76.75,33.45 | 77.3,20.4 U24.47 | J3.P$9 2.88,33.48 2.88,32.92 | 2.34,19.72 J5.P$3 2.62,20.37 | C17.1 C2.1
  Top 0.8: 76.75,33.45 77.23,33.45 78,34.22 U24.1 | U24.1 78,32.7 76.85,31.55 | U24.38 78,19.69 77.3,20.4 | U24.38 78,15.4 77.5,14.9 | 76.68,43.58 77.25,43.58 78,42.82 U24.1 | U24.38 78,11.3 | LED1.- 2.88,30.42 2.88,32.92
  other vias: 38.87,43.47 3.54,3.46 20.52,49.55 58.76,35.38 58.49,39.19 60.71,39.23 3.49,50.54 82.24,3.51 82.24,50.49 51.57,51.32 75.02,25.62 75.02,27.62 75.92,31.47 49.22,7.07 72.57,19.87 69.37,21.02 22.88,8.65 23.47,6.72 16.98,10.63 30.07,12.32 9.78,14.01 10.4,10.42 23.57,5.17 18.72,32.02 12.72,35.27 52.67,32.69 47.12,36.67 9.07,43.46 11.99,24.31 39.87,5.01 13.43,43.47 69.37,51.22 54.82,47.32 10.85,47.38 37.22,46.97 14.22,33.77 62.42,47.17 13.52,45.87 76.87,12.57 33.32,51.42 70.27,29.97 63.07,37.67 41.52,7.12 72.77,40.67 62.42,45.52 38.78,41.12 72.57,29.97 22.55,23.49 13.4,35.92 28.96,33.31 21.63,42.17 22.83,19.72 25.99,14.39 23.58,3.77 8.61,20.37 12.11,31.49 58.33,15.92 30.13,13.42 10.67,12.18 30.11,14.5 45.23,7.12 16.93,24.37 37.93,7.32 12.02,26.67 8.93,29.78 22.9,13.92 25.08,13.97 56.28,44.42 34.58,10.82 30.08,11.12 56.18,40.67 11.97,21.22 12.02,28.15 70.23,16.07 61.83,15.87 60.38,14.42 60.48,10.27 19.6,5.98 11.32,14.27 10.42,15.23 34.53,12.87 37.78,13.42 38.48,12.22 15.38,31.1 20.02,32.15 28.98,37.92 12.26,42.09 15.92,45.92 9.16,48.82 56.52,36.77 72.32,46.97 74.07,45.07 75.42,45.07 76.67,45.07 76.63,33.47 70.77,37.52 74.57,37.52 53.77,24.01 61.77,10.27 52.7,5.55 50.68,5.55 31.62,4.77 18.17,24.62 30.28,10.22 29.23,19.22 32.33,19.27 52.09,19.29 12.38,13.5 8.55,28.36 8.66,32.75 12.18,32.56 11.28,32.47 25.28,10.67 74.92,29.97 75.02,23.27 46.18,38.27 9.25,9.38 8.85,10.96 16.14,13.93 16.18,42.42 9.07,45.06 17.37,48.21 18.32,42.46 41.67,5.01 23.53,8 40.21,39.8 8.59,21.37 16.36,49.44 11.05,43.6 73.32,19.32 76.32,20.02 75.07,21.57 56.93,14.47 8.97,12.82 11.8,11.79 43.71,36.46 28.76,25.91 30.45,21.62 29.02,28.02 11,45.05 42.1,38.4 9.04,46.76 10.23,42.02 43.72,38.17 51.62,39.42 49.67,39.42 67.82,37.17 67.72,39.62 16.12,44.11 23.01,45.45 8.59,22.89 33.97,27.85 35.91,26.84 68.8,14.89 70.57,14.89 17.62,32.07
  pour Bottom: 77.6,52.08 77.6,1.9 8.17,1.9 8.17,52.08
  pour Top: -0.05,54.1 85.88,54.1 85.88,47.72 78.49,47.72 78.49,6.39 85.8,6.39 85.8,0 -0.05,0
IN-
  Top 0.254: R37.1 74.93,7.87 | 74.93,7.87 73.24,7.87 U2.4 | R22.2 74.93,6.73 74.93,7.87
IO0_BOOT  (via drill 0.35)
  Top 0.254: U24.25 61.49,28.83 v61.69,29.03 | v25.2,44.15 25.2,50.1 24.15,51.15 16.23,51.15 14.56,49.48 K1.2 | Q10.3 40.37,37.82 v40.57,38.02
  Bottom 0.254: v61.69,29.03 49.56,29.03 v40.57,38.02 34.44,44.15 v25.2,44.15
IO2_TFT_RS  (via drill 0.35)
  Top 0.254: v50.68,23.07 51.03,23.07 53.35,20.75 U24.24
  Bottom 0.254: v50.68,23.07 50.53,23.21 25.33,23.21 J1.P$4
IO5_TF_CS
  Top 0.254: R67.2 40.88,18.53 40.88,17.47 42.13,16.22 SD1.2 42.13,14.46 43.19,13.4 63.05,13.4 66.57,16.92 U24.29
IO12_TFT_SDO/TP_OUT  (via drill 0.35)
  Top 0.254: v64.03,21.66 63.95,21.74 63.95,31.3 61.49,33.76 U24.14 60.07,33.84 R2.1 | U3.12 18.97,20.35 v18.97,22.03
  Bottom 0.254: v64.03,21.66 58.08,21.66 53.5,17.07 21.59,17.07 18.97,19.7 v18.97,22.03
IO13_TFT_SDI/TP_DIN  (via drill 0.35)
  Top 0.254: R29.1 43.48,20.14 v43.48,24.98 56.65,24.98 58.21,26.55 58.21,30.07 59.05,30.91 U24.16 | U3.14 20.26,22.66 v20.5,22.9
  Bottom 0.254: v43.48,24.98 43.35,24.84 J1.P$6 22.44,24.84 v20.5,22.9
IO14_TFT_CLK/TP_CLK  (via drill 0.35)  (2 unrouted)
  Top 0.254: U24.13 62.76,33.61 64.66,31.71 v64.66,24.72 | v44.66,22.48 44.69,22.45 44.69,20.05 | v22.8,21.05 22.07,20.32 U3.16
  Bottom 0.254: v64.66,24.72 v64.65,24.73 56.28,24.73 53.3,21.75 50.6,21.75 49.87,22.48 v44.66,22.48 44.63,22.44 J1.P$3 | v22.8,21.05 22.8,21.97 23.24,22.41 25.08,22.41
IO15_TFT_CS  (via drill 0.35)
  Top 0.254: v52.18,23.82 53.98,22.02 U24.23
  Bottom 0.254: J1.P$5 51.96,24.04 v52.18,23.82
IO16_RXD2  (via drill 0.35)
  Top 0.254: U24.27 63.84,17.86 63.84,18.26 62.29,19.81 v62.29,25.83 | v32.18,41.27 31.28,42.17 J10.1
  Bottom 0.254: v62.29,25.83 47.62,25.83 v32.18,41.27
IO17_TXD2  (via drill 0.35)  (1 unrouted)
  Top 0.254: U24.28 65.21,17.76 65.21,18.63 63.22,20.62 v63.22,26.87 | v33.35,41.87 33.3,41.92 33.3,43.85
  Bottom 0.254: v33.35,41.87 48.35,26.87 v63.22,26.87
IO18_TF_SPI_CLK
  Top 0.254: U24.30 67.84,16.57 63.04,11.77 40.08,11.77 38.83,13.02 SD1.5
IO19_TF_SPI_MISO
  Top 0.254: R24.2 35.53,18.53 35.53,17.47 36.63,16.37 SD1.7 36.63,12.89 38.25,11.28 63.47,11.28 69.11,16.92 U24.31
IO21_SCL  (via drill 0.35)  (1 unrouted)
  Top 0.254: 49.53,35.59 v49.53,37.15 48.74,37.93 J6.1 | U24.33 71.65,21.7 v70.25,23.1
  Bottom 0.254: v70.25,23.1 70.25,27.13 67.16,30.22 52.36,30.22 49.53,33.05 v49.53,37.15
IO22_SDA  (via drill 0.35)
  Top 0.254: U24.36 75.46,19.49 71.95,23 v71.9,23 | J6.2 50.88,44.11 v50.88,37.23 R27.1
  Bottom 0.254: v71.9,23 71.9,27.1 67.9,31.1 52.75,31.1 50.88,32.98 v50.88,37.23
IO23_TF_SPI_MOSI  (via drill 0.35)
  Top 0.254: R23.2 39.58,17.57 41.03,16.12 SD1.3 41.03,13.65 42.23,12.46 62.59,12.46 v62.61,12.48 | U24.37 76.73,14.01 75.21,12.48 v75.06,12.48
  Bottom 0.254: v75.06,12.48 v62.61,12.48
IO25_PROT_A/D  (via drill 0.35)
  Top 0.254: v66.53,33.8 66.57,33.84 U24.10 66.57,40.68 66.05,41.2 66.05,44.12 J7.1 | R18.1 53.92,32.93 54.19,32.66 v55.19,32.66
  Bottom 0.254: v66.53,33.8 65.93,33.2 56.23,33.2 55.69,32.66 v55.19,32.66
IO26_SPEAK  (via drill 0.35)
  Top 0.254: U24.11 65.3,33.37 65.9,32.77 65.9,20.78 66.89,19.79 68.29,19.79 v68.44,19.64 | v72.02,16.15 72.04,16.13 72.04,13.87 R12.1
  Bottom 0.254: v72.02,16.15 72.02,16.2 68.58,19.64 v68.44,19.64
IO27_LCD_BLK_CTR  (via drill 0.35)
  Top 0.254: U24.12 64.03,33.94 65.4,32.57 v65.4,19.52 | v15.9,26.72 14.51,26.72 Q6.1 14.42,26.62 R38.1
  Bottom 0.254: v65.4,19.52 59.36,19.52 55.12,15.28 20.66,15.28 15.9,20.04 v15.9,26.72
IO32_PROT_A/D  (via drill 0.35)
  Top 0.254: v68.95,33.25 69.11,33.41 U24.8 69.11,40.34 68.22,41.23 J7.2 | v57.85,32.15 56.85,32.15 55.35,33.65 R1.1
  Bottom 0.254: v68.95,33.25 67.85,32.15 v57.85,32.15
IO33_TP_CS  (via drill 0.35)
  Top 0.254: U24.9 67.84,33.37 66.69,32.22 66.69,22.39 v66.72,22.37 | U3.15 20.9,19.34 22.04,18.2 v22.32,18.2
  Bottom 0.254: v66.72,22.37 66.3,22.78 57.06,22.78 52.48,18.2 v22.32,18.2
IO36_TP_IRQ  (via drill 0.35)
  Top 0.254: v67.5,20.6 67.5,30.4 69.62,32.52 72.24,32.52 74.19,34.47 U24.4 | U3.11 18.36,21.24 v17.6,22 16.9,22 16,21.1 16,20.09 15.16,19.26 R10.1
  Bottom 0.254: v67.5,20.6 58.75,20.6 54.35,16.2 21.19,16.2 17.6,19.79 v17.6,22
N$1
  Top 0.254: LED1.+ 3.34,28.39
  Top 0.8: R3.1 3.37,28.46 LED1.+
N$2
  Top 0.254: R7.2 13.27,22.1 15.04,23.87 Q6.3
N$3
  Top 0.254: R12.2 71.44,11.79 70.17,13.06 R19.1 C46.2
N$4
  Top 0.254: U3.7 17.72,27.2 16.72,28.21 R35.2
N$5
  cutout Top: 76.56,5.13 76.89,5.13 76.89,4.29 76.56,4.29
N$6
  Top 0.8: U26.5 4.1,26.07 R9.1
N$8
  Top 0.8: L4.1 27.31,2.42 U1.3
N$12  (via drill 0.35)
  Top 0.254: R7.1 14.67,22.29 15.66,23.27 19.74,23.27 19.85,23.39 19.85,24.2 v19.6,24.45
  Bottom 0.254: 25.31,29.73 J1.P$11 25.29,28.86 23.49,28.86 19.6,24.97 v19.6,24.45
  Bottom 0.5: J1.P$14 J1.P$13 25.31,29.73 | J1.P$12 J1.P$11
N$14
  Top 0.254: J3.B5 9.94,36.3 12.92,33.33 12.92,29.71 R33.1
N$16  (1 unrouted)
  Top 0.254: 8.11,39.29 10.25,39.29 R34.2
N$17
  Top 0.8: R25.1 9.27,4.16 R6.2 11.62,4.16 Q3.1
N$20
  Top 0.254: U1.5 21.76,6.19 21.76,10.27 R21.1 R20.2
N$26
  Top 0.254: C51.2 67.57,11.08 68,10.65 69.7,10.65 70.17,11.12 R19.2 70.17,11.25 71.83,9.59 76.26,9.59 77.6,8.25 77.6,6.21 C14.1
N$29
  Top 0.254: C14.2 76.43,6.56 R22.1
N$32
  Top 0.254: R75.1 32.04,35.23 34.03,35.23 Q9.1
N$38
  Top 0.254: Q10.1 33.32,38.06 31.62,38.06 30.55,36.99 R74.1
N$40  (via drill 0.35)
  Top 0.254: R72.2 72.74,11.19 v72.11,10.56 | v22.25,38.85 22.23,38.87 U6.2
  Bottom 0.254: v72.11,10.56 70.86,9.31 24.54,9.31 14.65,19.2 14.65,31.39 22.11,38.85 v22.25,38.85
N$42  (via drill 0.35)
  Top 0.254: R71.2 74.07,10.92 v73.7,10.55 | v20.82,39.14 20.82,40.3 U6.3
  Bottom 0.254: v73.7,10.55 73.65,10.55 71.6,8.5 24.15,8.5 13.82,18.83 13.82,31.98 20.82,38.97 v20.82,39.14
N$47
  Top 0.254: R16.2 42.08,18.58 42.08,17.62 43.23,16.47 SD1.1
N$48
  Top 0.254: R17.2 34.33,18.45 34.33,17.12 35.53,15.92 SD1.8
RTS  (via drill 0.35)
  Top 0.254: Q9.2 33.69,33.77 v32.88,33.77 32.72,33.93 31.37,33.93 30.55,34.75 R74.2 | U6.14 v20.96,34.2 v20.95,34.19
  Bottom 0.254: v32.88,33.77 32.88,35.02 32.28,35.62 22.38,35.62 v20.95,34.19
TFT_RESET  (via drill 0.35)
  Top 0.254: R5.1 49.07,18.59 C28.1 46.23,20.01 R8.1 46.23,21.05 v46.3,21.13
  Bottom 0.254: v46.3,21.13 45.95,20.77 28.37,20.77 27.43,21.72 25.38,21.72 J1.P$2
TP_X+  (via drill 0.35)
  Top 0.254: U3.2 20.9,26.83 21.94,27.87 C18.2 22.07,29.57 v22.8,30.3
  Bottom 0.254: J1.P$15 23.35,32.04 22.8,31.49 v22.8,30.3
TP_X-  (via drill 0.35)
  Top 0.254: C20.2 19.38,29.55 19.38,27.82 v19.62,27.57 v19.63,27.57 U3.4
  Bottom 0.254: J1.P$17 23.42,33.64 21.3,31.52 21.3,28.17 20.6,27.47 19.72,27.47 v19.62,27.57
TP_Y+  (via drill 0.35)
  Top 0.254: C19.2 20.66,28.48 v20.54,28.48 20.54,27.34 20.26,27.07 U3.3
  Bottom 0.254: v20.54,28.48 20.54,31.64 23.4,34.5 25.25,34.5 J1.P$18
TP_Y-  (via drill 0.35)  (1 unrouted)
  Top 0.254: U3.5 18.99,26.86 18.07,27.78 v18.07,28.33 18.07,29.66
  Bottom 0.254: J1.P$16 23.38,32.84 21.9,31.36 21.9,28.06 20.64,26.79 19.06,26.79 18.07,27.78 v18.07,28.33
UART0_RXD0
  Top 0.254: U24.34 73.24,17.35 73.24,13.77 R72.1
UART0_TXD0
  Top 0.254: U24.35 74.54,17.32 74.54,14.07 74.07,13.59 R71.1
USB_D+
  Top 0.254: R32.2 12.39,37.19 12.39,37.21 12.98,37.8 16.5,37.8 18.42,39.72 U6.5
USB_D-
  Top 0.254: R11.2 12.38,38.45 16.25,38.45 17.15,39.35 U6.6
VBUS  (via drill 0.35)  (5 unrouted)
  Top 0.5: 6.96,40.51 7.02,40.45
  Top 0.6: 7.93,35.65 6.9,35.65 | 7.02,40.45 7.78,40.45 | 8.24,35.65 9.2,35.65
  Top 0.65: 6.9,35.65 5.75,36.8 5.75,39.3 6.96,40.51
  Top 0.7: 9.2,35.65 10.09,34.76
  Top 0.8: C27.1 U26.4 7.21,26.29 C25.2 9.96,26.29 10.09,26.16 | 14.3,15.79 14.91,15.17 v14.91,14.88 | v9.37,7.9 9.26,7.79 R25.2
  Top 1: D3.1 16.25,15.79 14.3,15.79 10.09,20 10.09,26.16 10.09,34.76
  Bottom 0.8: v14.91,14.88 14.91,13.44 v9.37,7.9
VIN
  Top 0.3: 22.26,4.82 20.38,2.94
  Top 0.5: U1.1 20.38,2.94 | 22.26,4.82 U1.4
  Top 0.65: C42.2 18.11,7 D3.2 | C6.2 17.96,4.14 C42.2 | C42.2 18.51,4.29 U1.1
  Top 0.8: Q3.2 15.25,4.14 C6.2 | D1.C 18.88,8.15 D3.2
VO1  (via drill 0.5)
  Top 0.254: J8.P$1 55.01,7.25 | U2.5 67.42,7.39 | 76.61,7.92 R37.2
  Top 0.5: v53.9,7.25 55.01,7.25 | 67.42,7.39 v65.67,7.39 | U2.5 68.88,8.84 75.7,8.84 76.61,7.92
  Bottom 0.5: v65.67,7.39 65.57,7.29 53.94,7.29 v53.9,7.25
VO2  (via drill 0.5)  (1 unrouted)
  Top 0.254: U2.8 67.09,3.61 | 56.99,7.19 57.15,7.35
  Top 0.5: 67.09,3.61 65.68,5.02 v65.68,5.27 | v56.99,5.34 56.99,7.19
  Bottom 0.5: v56.99,5.34 57.06,5.27 v65.68,5.27

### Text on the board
tPlace: GND | IO25 | IO32 | 3V3 | GND | IO16_RXD2 | IO17_TXD2 | 3V3 | IO21_SCL | IO22_SDA | 3V3 | GND | www.elecrow.com | + | V2.0 | IO26-SPK | - | VON- | VOP+
tNames: GND | 5V
tStop: ESP32 Display-2.8 Inch | SKU:DIS04028H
